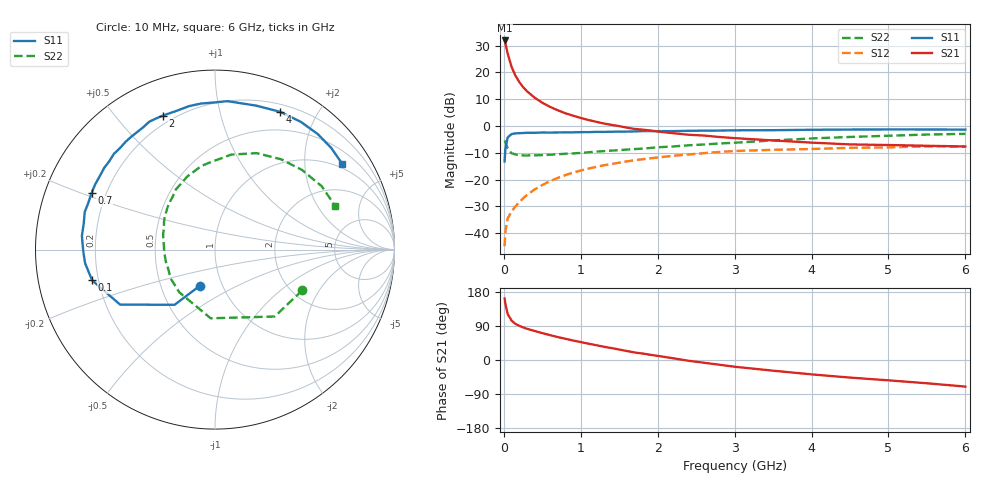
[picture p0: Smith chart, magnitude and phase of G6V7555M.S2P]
! SIEMENS Small Signal Semiconductors
! BFG193
! Si NPN RF Bipolar Junction Transistor in SOT223
! VCE = 0.75 V  IC = 55 mA
! Common Emitter S-Parameters:  August  1996
# GHz  S  MA  R  50
!  f  S11  S21  S12  S22
! GHz  MAG  ANG  MAG  ANG  MAG  ANG  MAG  ANG
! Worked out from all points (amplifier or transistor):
!   36 points, 10 MHz to 6 GHz, reference 50 ohm
!   highest |S21| = 31.9 dB at 10 MHz (marker M1)
!   |S21| within 3 dB of that: start of sweep to 35.08 MHz
!   unconditionally stable (mu >= 1): start of sweep to 17.1 MHz; 148.8 MHz to end of sweep
!   at 250 MHz: K = 1.14, MAG = 18.5 dB, |S12| = -27.0 dB
!   at 1.4 GHz: K = 1.20, MAG = 4.6 dB, |S12| = -14.2 dB
!   at 6 GHz: K = 1.08, MAG = -1.7 dB, |S12| = -7.7 dB
!   S11 on the Smith chart (normalised r, x): 10 MHz: 0.78, -0.33; 100 MHz: 0.17, -0.12; 700 MHz: 0.15, +0.21; 2 GHz: 0.16, +0.67; 4 GHz: 0.28, +1.54; 6 GHz: 0.86, +3.05
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0.01  0.2179 -112.7  39.5 162.3  0.0057 69.9  0.5369 -25.0
0.02  0.3811 -126.2  34.93 147.9  0.0108 64.0  0.4993 -48.3
0.05  0.6112 -149.9  22.44 121.1  0.0187 52.3  0.3835 -93.6
0.1  0.7059 -166.0  12.77 104.1  0.0254 52.6  0.3101 -129.8
0.15  0.7276 -174.0  8.717 95.4  0.0313 54.9  0.2949 -147.3
0.2  0.7332 -178.7  6.637 90.2  0.0379 58.4  0.2821 -156.8
0.25  0.7387 177.4  5.318 86.0  0.0445 59.9  0.282 -164.8
0.3  0.7454 174.1  4.462 82.5  0.0515 61.8  0.2816 -169.4
0.4  0.7456 168.8  3.379 76.6  0.0652 62.6  0.2834 -177.9
0.5  0.7554 163.9  2.717 70.9  0.079 62.0  0.2853 175.9
0.6  0.7524 159.5  2.276 65.7  0.0934 60.8  0.2903 171.2
0.7  0.7565 155.4  1.964 60.5  0.1069 59.2  0.2964 166.9
0.9  0.7616 147.3  1.557 51.4  0.1345 54.9  0.3074 158.2
1.1  0.7674 140.3  1.291 43.1  0.1601 50.7  0.3232 151.5
1.6  0.7856 123.3  0.93 23.7  0.2184 38.0  0.3627 135.0
2  0.8012 111.2  0.789 10.9  0.2577 27.6  0.4 123.0
2.2  0.8018 105.8  0.733 4.6  0.2773 22.5  0.4141 116.9
3.5  0.8344 74.0  0.537 -28.2  0.3588 -11.0  0.5371 80.3
4  0.849 64.7  0.489 -37.9  0.3715 -20.5  0.5856 66.6
4.5  0.8575 56.1  0.453 -46.4  0.391 -30.2  0.6237 53.8
5.5  0.8605 41.2  0.427 -61.4  0.4158 -51.9  0.6915 30.7
6  0.855 34.0  0.414 -70.2  0.4113 -64.2  0.713 19.7
